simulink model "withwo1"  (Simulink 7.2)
settings: Solver=ode45  StartTime=0.0  StopTime=15  MaxStep=0.05  RelTol=1e-3
InitFcn:
  | init_withworth;
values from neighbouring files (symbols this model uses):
  L1 = 2    [init_withworth.m]    (also in init_ctyrkloub.m = 3; init_klik.m = 1.5)
  L2 = 5    [init_withworth.m]    (also in init_ctyrkloub.m; init_klik.m = v/sin(uhel3))
  omega = 0.5    [init_withworth.m]    (also in init_ctyrkloub.m = 1; init_klik.m = 5)
undefined symbols (not defined in the file or in its folder): deg, kg, m, N, rad, s
libraries: mblibv1 x14, simulink x1

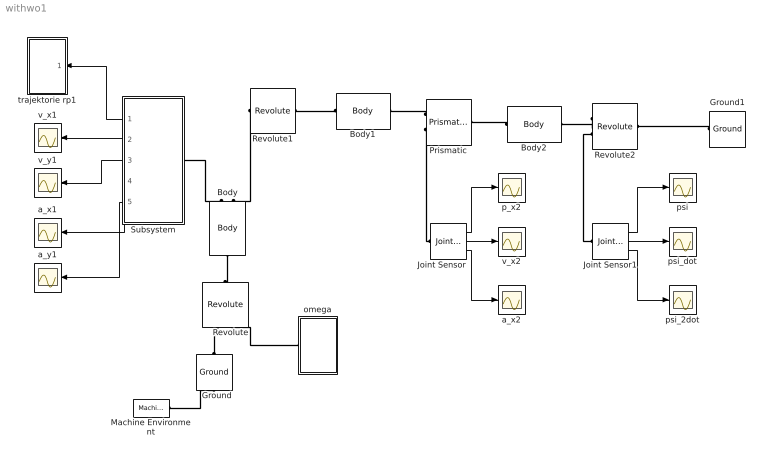
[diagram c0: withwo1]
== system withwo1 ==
  Body : mblibv1/Bodies/Body  Orientation=up  DialogController=MECH.DynMechDlgSource  PhysicalDomain=mechanical  SubClassName=Unknown  LeftPortType=workingframe  RightPortType=workingframe  LConnTagsString=CS1  RConnTagsString=CS3|CS2  UpdateFromCAD=off  DialogClass=MechanicalBodyBlock  Mass=1  MassUnits=kg  InertiaUnits=kg*m^2  Inertia=eye(3)  Shape=Cylinder  ShapeDims=[1 1]  ShapeUnits=m  ShapeUse=false  Density=1  DensityUnits=kg/m^3  DensityUse=false  GraphicsMode=MACHINE_DEFAULT  BodyColorSelMode=MACHINE_DEFAULT  BodyColor=[1 0 0]  AttachedToCS=CG  CG=Left$CG$[L1/2 0 0]$CS1$CS1$m$[0 0 pi/3]$Euler X-Y-Z$rad$WORLD$false$none  WorkingFrames=Right$CS3$[0 0 0]$CS2$CS2$m$[0 0 pi/3]$Euler X-Y-Z$rad$WORLD$true$none#Left$CS1$[0 0 0]$Adjoining$Adjoining$m$[0 0 pi/3]$Euler X-Y-Z$rad$WORLD$true$none#Right$CS2$[L1 0 0]$CS1$CS1$m$[0 0 pi/3]$Euler X-Y-Z$rad$WORLD$true$none  CGPos=[L1/2 0 0]  CGRot=[0 0 pi/3]  CS0Pos=[]  CS0Rot=[]  CS1Pos=[0 0 0]  CS1Rot=[0 0 pi/3]  CS2Pos=[L1 0 0]  CS2Rot=[0 0 pi/3]  CS3Pos=[0 0 0]  CS3Rot=[0 0 pi/3]  CS4Pos=[]  CS4Rot=[]  CS5Pos=[]  CS5Rot=[]  CS6Pos=[]  CS6Rot=[]  CS7Pos=[]  CS7Rot=[]  CS8Pos=[]  CS8Rot=[]  CS9Pos=[]  CS9Rot=[]  CS10Pos=[]  CS10Rot=[]  CS11Pos=[]  CS11Rot=[]  CS12Pos=[]  CS12Rot=[]  CS13Pos=[]  CS13Rot=[]  CS14Pos=[]  CS14Rot=[]  CS15Pos=[]  CS15Rot=[]  CS16Pos=[]  CS16Rot=[]  CS17Pos=[]  CS17Rot=[]  CS18Pos=[]  CS18Rot=[]  CS19Pos=[]  CS19Rot=[]  CS20Pos=[]  CS20Rot=[]
  Body1 : mblibv1/Bodies/Body  DialogController=MECH.DynMechDlgSource  PhysicalDomain=mechanical  SubClassName=Unknown  LeftPortType=workingframe  RightPortType=workingframe  LConnTagsString=CS1  RConnTagsString=CS2  UpdateFromCAD=off  DialogClass=MechanicalBodyBlock  Mass=1  MassUnits=kg  InertiaUnits=kg*m^2  Inertia=eye(3)  Shape=Cylinder  ShapeDims=[1 1]  ShapeUnits=m  ShapeUse=false  Density=1  DensityUnits=kg/m^3  DensityUse=false  GraphicsMode=MACHINE_DEFAULT  BodyColorSelMode=MACHINE_DEFAULT  BodyColor=[1 0 0]  AttachedToCS=CG  CG=Left$CG$[0 0 0]$CS1$CS1$m$[0 0 0]$Euler X-Y-Z$rad$CS1$false$none  WorkingFrames=Left$CS1$[0 0 0]$Adjoining$Adjoining$m$[0 0 3*pi/2]$Euler X-Y-Z$rad$Adjoining$true$none#Right$CS2$[0 0 0]$CS1$CS1$m$[0 0 0]$Euler X-Y-Z$rad$CS1$true$none  CGPos=[0 0 0]  CGRot=[0 0 0]  CS0Pos=[]  CS0Rot=[]  CS1Pos=[0 0 0]  CS1Rot=[0 0 3*pi/2]  CS2Pos=[0 0 0]  CS2Rot=[0 0 0]  CS3Pos=[]  CS3Rot=[]  CS4Pos=[]  CS4Rot=[]  CS5Pos=[]  CS5Rot=[]  CS6Pos=[]  CS6Rot=[]  CS7Pos=[]  CS7Rot=[]  CS8Pos=[]  CS8Rot=[]  CS9Pos=[]  CS9Rot=[]  CS10Pos=[]  CS10Rot=[]  CS11Pos=[]  CS11Rot=[]  CS12Pos=[]  CS12Rot=[]  CS13Pos=[]  CS13Rot=[]  CS14Pos=[]  CS14Rot=[]  CS15Pos=[]  CS15Rot=[]  CS16Pos=[]  CS16Rot=[]  CS17Pos=[]  CS17Rot=[]  CS18Pos=[]  CS18Rot=[]  CS19Pos=[]  CS19Rot=[]  CS20Pos=[]  CS20Rot=[]
  Body2 : mblibv1/Bodies/Body  DialogController=MECH.DynMechDlgSource  PhysicalDomain=mechanical  SubClassName=Unknown  LeftPortType=workingframe  RightPortType=workingframe  LConnTagsString=CS1  RConnTagsString=CS2  UpdateFromCAD=off  DialogClass=MechanicalBodyBlock  Mass=1  MassUnits=kg  InertiaUnits=kg*m^2  Inertia=eye(3)  Shape=Cylinder  ShapeDims=[1 1]  ShapeUnits=m  ShapeUse=false  Density=1  DensityUnits=kg/m^3  DensityUse=false  GraphicsMode=MACHINE_DEFAULT  BodyColorSelMode=MACHINE_DEFAULT  BodyColor=[1 0 0]  AttachedToCS=CG  CG=Left$CG$[L2/2 0 0]$CS1$CS1$m$[0 0 0]$Euler X-Y-Z$deg$CS1$false$none  WorkingFrames=Left$CS3$[-L2/2 0 0]$CS1$CS1$m$[0 0 0]$Euler X-Y-Z$deg$CS1$false$none#Left$CS1$[0 0 0]$Adjoining$Adjoining$m$[0 0 0]$Euler X-Y-Z$deg$Adjoining$true$none#Right$CS2$[L2 0 0]$CS1$CS1$m$[0 0 0]$Euler X-Y-Z$deg$CS1$true$none  CGPos=[L2/2 0 0]  CGRot=[0 0 0]  CS0Pos=[]  CS0Rot=[]  CS1Pos=[0 0 0]  CS1Rot=[0 0 0]  CS2Pos=[L2 0 0]  CS2Rot=[0 0 0]  CS3Pos=[-L2/2 0 0]  CS3Rot=[0 0 0]  CS4Pos=[]  CS4Rot=[]  CS5Pos=[]  CS5Rot=[]  CS6Pos=[]  CS6Rot=[]  CS7Pos=[]  CS7Rot=[]  CS8Pos=[]  CS8Rot=[]  CS9Pos=[]  CS9Rot=[]  CS10Pos=[]  CS10Rot=[]  CS11Pos=[]  CS11Rot=[]  CS12Pos=[]  CS12Rot=[]  CS13Pos=[]  CS13Rot=[]  CS14Pos=[]  CS14Rot=[]  CS15Pos=[]  CS15Rot=[]  CS16Pos=[]  CS16Rot=[]  CS17Pos=[]  CS17Rot=[]  CS18Pos=[]  CS18Rot=[]  CS19Pos=[]  CS19Rot=[]  CS20Pos=[]  CS20Rot=[]
  Ground : mblibv1/Bodies/Ground  Orientation=up  DialogController=MECH.DynMechDlgSource  SystemSampleTime=-1  UpdateFromCAD=off  LeftPortType=env  RightPortType=workingframe  PhysicalDomain=Mechanical  DialogClass=GroundBlock  CoordPosition=[0 0 0]  CoordPositionUnits=m  StateVectorMgrId=2  MachineId=[3 0]  ShowEnvPort=on
  Ground1 : mblibv1/Bodies/Ground  Orientation=left  DialogController=MECH.DynMechDlgSource  SystemSampleTime=-1  UpdateFromCAD=off  LeftPortType=env  RightPortType=workingframe  PhysicalDomain=Mechanical  DialogClass=GroundBlock  CoordPosition=[L1*cos(pi/3)+L2*cos(pi/6) L1*sin(pi/3)-L2*sin(pi/6) 0]  CoordPositionUnits=m  StateVectorMgrId=-1  MachineId=[0 0]  ShowEnvPort=off
  Joint Sensor : mblibv1/Sensors &  Actuators/Joint Sensor  DialogController=MECH.DynMechDlgSource  SystemSampleTime=-1  UpdateFromCAD=off  PhysicalDomain=Mechanical  PortType=blob  Muxed=off  Pose=off  Angle=on  AngleUnits=deg  ArcVelocity=off  ArcVelocityUnits=deg/s  ArcAcceleration=off  ArcAccelerationUnits=deg/s^2  CoordPosition=on  CoordPositionUnits=m  Velocity=on  VelocityUnits=m/s  Acceleration=on  AccelerationUnits=m/s^2  Quaternion=on  QuaternionDT=off  QuaternionDDT=off  QuaternionUnits=off  OutputVector=[1]  ActiveIO=on  Width=3  DialogClass=MechanicalSensorBlock  Primitive=P1  Force=off  ForceUnits=N  Torque=off  TorqueUnits=N*m  ReferenceFrame=Absolute (World)  ReactionSensedSide=Base  ReactionReferenceFrame=Absolute (World)  ReactionForce=off  ReactionForceUnits=N  ReactionMoment=off  ReactionMomentUnits=N*m
  Joint Sensor1 : mblibv1/Sensors &  Actuators/Joint Sensor  DialogController=MECH.DynMechDlgSource  SystemSampleTime=-1  UpdateFromCAD=off  PhysicalDomain=Mechanical  PortType=blob  Muxed=off  Pose=off  Angle=on  AngleUnits=rad  ArcVelocity=on  ArcVelocityUnits=rad/s  ArcAcceleration=on  ArcAccelerationUnits=rad/s^2  CoordPosition=on  CoordPositionUnits=m  Velocity=on  VelocityUnits=m/s  Acceleration=on  AccelerationUnits=m/s^2  Quaternion=on  QuaternionDT=off  QuaternionDDT=off  QuaternionUnits=off  OutputVector=[1]  ActiveIO=on  Width=3  DialogClass=MechanicalSensorBlock  Primitive=R1  Force=off  ForceUnits=N  Torque=off  TorqueUnits=N*m  ReferenceFrame=Absolute (World)  ReactionSensedSide=Base  ReactionReferenceFrame=Absolute (World)  ReactionForce=off  ReactionForceUnits=N  ReactionMoment=off  ReactionMomentUnits=N*m
  Machine Environment : mblibv1/Bodies/Machine Environment  DialogController=MECH.DialogSource  SystemSampleTime=-1  PortType=env  PhysicalDomain=Mechanical  DialogTemplateClass=MECH.MachineEnvironment  SyncWhenCopied=off  Gravity=[0 -9.81 0]  GravityUnits=m/s^2  GravityAsSignal=off  Dimensionality=Auto-detect  AnalysisType=Kinematics  LinearAssemblyTolerance=1e-3  LinearAssemblyToleranceUnits=m  AngularAssemblyTolerance=1e-3  AngularAssemblyToleranceUnits=rad  ConstraintSolverType=Stabilizing  ConstraintRelTolerance=1e-4  ConstraintAbsTolerance=1e-4  UseRobustSingularityHandling=off  RedundancyAnalysisToleranceType=Automatically select tolerance  RedundancyAnalysisTolerance=1e-14  StatePerturbationType=Fixed  PerturbationSize=1e-5  VisualizeMachine=on  BodyVisualizationType=Use model default body geometries  BodyColorSelMode=Use model default  DefaultBodyColor=[1 0 0]
  Prismatic : mblibv1/Joints/Prismatic  DialogController=MECH.DynMechDlgSource  PhysicalDomain=mechanical  SubClassName=Unknown  LeftPortType=blob  RightPortType=blob  LConnTagsString=__newl0|SA1  RConnTagsString=__newr0  UpdateFromCAD=off  NumSAPorts=1  CutJoint=off  MarkAsCut=off  Primitives=prismatic  PrimitiveProps=P1$Base$[-1 0 0]$prismatic  DialogClass=JointBlock  P1Axis=[-1 0 0]
  Revolute : mblibv1/Joints/Revolute  Orientation=up  DialogController=MECH.DynMechDlgSource  PhysicalDomain=mechanical  SubClassName=Unknown  LeftPortType=blob  RightPortType=blob  LConnTagsString=__newl0|SA1  RConnTagsString=__newr0  UpdateFromCAD=off  NumSAPorts=1  CutJoint=off  MarkAsCut=off  Primitives=prismatic  PrimitiveProps=R1$World$[0 0 1]$revolute  DialogClass=JointBlock  R1Axis=[0 0 1]
  Revolute1 : mblibv1/Joints/Revolute  DialogController=MECH.DynMechDlgSource  PhysicalDomain=mechanical  SubClassName=Unknown  LeftPortType=blob  RightPortType=blob  LConnTagsString=__newl0  RConnTagsString=__newr0  UpdateFromCAD=off  NumSAPorts=0  CutJoint=off  MarkAsCut=off  Primitives=prismatic  PrimitiveProps=R1$WORLD$[0 0 1]$revolute  DialogClass=JointBlock  R1Axis=[0 0 1]
  Revolute2 : mblibv1/Joints/Revolute  DialogController=MECH.DynMechDlgSource  PhysicalDomain=mechanical  SubClassName=Unknown  LeftPortType=blob  RightPortType=blob  LConnTagsString=__newl0|SA1  RConnTagsString=__newr0  UpdateFromCAD=off  NumSAPorts=1  CutJoint=off  MarkAsCut=off  Primitives=prismatic  PrimitiveProps=R1$World$[0 0 1]$revolute  DialogClass=JointBlock  R1Axis=[0 0 1]
  Subsystem : Subsystem  Orientation=left
  a_x1 : Scope
  a_x2 : Scope
  a_y1 : Scope
  omega : Subsystem  Orientation=left
  p_x2 : Scope
  psi : Scope
  psi_2dot : Scope
  psi_dot : Scope
  trajektorie rp1 : Subsystem  Orientation=left
  v_x1 : Scope
  v_x2 : Scope
  v_y1 : Scope
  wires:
  Joint Sensor/1 -> p_x2/1
  Joint Sensor/2 -> v_x2/1
  Joint Sensor/3 -> a_x2/1
  Subsystem/1(Out1) -> trajektorie rp1/1(In1)
  Subsystem/2(Out2) -> v_x1/1
  Subsystem/3(Out3) -> v_y1/1
  Subsystem/4(Out4) -> a_x1/1
  Subsystem/5(Out5) -> a_y1/1
  Joint Sensor1/1 -> psi/1
  Joint Sensor1/2 -> psi_dot/1
  Joint Sensor1/3 -> psi_2dot/1
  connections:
  Ground/RConn1 -- Revolute/LConn1
  Body/LConn1 -- Revolute/RConn1
  Revolute1/LConn1 -- Body/RConn2
  Body1/LConn1 -- Revolute1/RConn1
  Prismatic/LConn1 -- Body1/RConn1
  Body2/LConn1 -- Prismatic/RConn1
  Ground1/RConn1 -- Revolute2/RConn1
  Revolute2/LConn1 -- Body2/RConn1
  Subsystem/LConn1 -- Body/RConn1
  omega/RConn1 -- Revolute/LConn2
  Joint Sensor/LConn1 -- Prismatic/LConn2
  Machine Environment/RConn1 -- Ground/LConn1
  Joint Sensor1/LConn1 -- Revolute2/LConn2

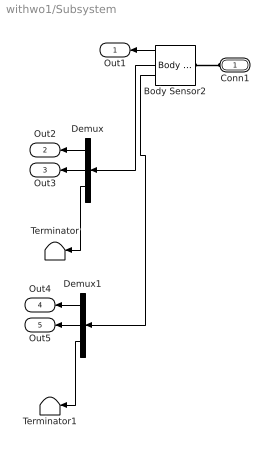
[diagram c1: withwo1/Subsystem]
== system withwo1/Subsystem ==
  Body Sensor2 : mblibv1/Sensors &  Actuators/Body Sensor  Orientation=left  DialogController=MECH.DynMechDlgSource  SystemSampleTime=-1  UpdateFromCAD=off  PhysicalDomain=Mechanical  PortType=blob  Muxed=off  Pose=off  Angle=on  AngleUnits=deg  ArcVelocity=off  ArcVelocityUnits=deg/s  ArcAcceleration=off  ArcAccelerationUnits=deg/s^2  CoordPosition=on  CoordPositionUnits=m  Velocity=on  VelocityUnits=m/s  Acceleration=on  AccelerationUnits=m/s^2  Quaternion=on  QuaternionDT=off  QuaternionDDT=off  QuaternionUnits=off  OutputVector=[1]  ActiveIO=on  Width=9  DialogClass=MechanicalSensorBlock  ReferenceFrame=Absolute (World)
  Demux : Demux  Orientation=left  Outputs=3
  Demux1 : Demux  Orientation=left  Outputs=3
  Terminator : Terminator
  Terminator1 : Terminator
  Conn1 : PMIOPort  Orientation=left  Port=1  Side=Left
  Out1 : Outport  Orientation=left
  Out2 : Outport  Orientation=left  Port=2
  Out3 : Outport  Orientation=left  Port=3
  Out4 : Outport  Orientation=left  Port=4
  Out5 : Outport  Orientation=left  Port=5
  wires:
  Demux/3 -> Terminator/1
  Body Sensor2/2 -> Demux/1
  Demux1/3 -> Terminator1/1
  Body Sensor2/3 -> Demux1/1
  Body Sensor2/1 -> Out1/1
  Demux/1 -> Out2/1
  Demux/2 -> Out3/1
  Demux1/1 -> Out4/1
  Demux1/2 -> Out5/1
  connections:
  Conn1/RConn1 -- Body Sensor2/LConn1

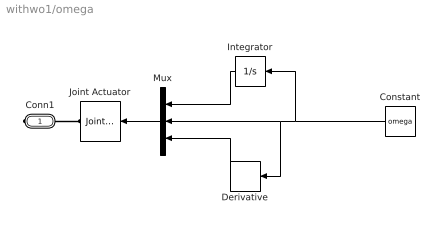
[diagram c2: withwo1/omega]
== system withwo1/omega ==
  Constant : Constant  Orientation=left  Value=omega  OutDataType=sfix(16)  OutScaling=2^0
  Derivative : Derivative  Orientation=left
  Integrator : Integrator  Orientation=left
  Joint Actuator : mblibv1/Sensors &  Actuators/Joint Actuator  Orientation=left  DialogController=MECH.DynMechDlgSource  SystemSampleTime=-1  UpdateFromCAD=off  PhysicalDomain=Mechanical  PortType=blob  ActuationStyle=Motion  AngleUnits=rad  ArcVelocityUnits=rad/s  ArcAccelerationUnits=rad/s^2  CoordPositionUnits=m  VelocityUnits=m/s  AccelerationUnits=m/s^2  ForceUnits=N  TorqueUnits=N*m  ActiveIO=on  Width=3  DialogClass=MechanicalActuatorBlock  Primitive=R1  ReferenceFrame=Absolute (World)
  Mux : Mux  Orientation=left  Inputs=3
  Conn1 : PMIOPort  Port=1  Side=Right
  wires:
  Constant/1 -> Derivative/1, Mux/2, Integrator/1
  Mux/1 -> Joint Actuator/1
  Integrator/1 -> Mux/1
  Derivative/1 -> Mux/3
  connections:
  Conn1/RConn1 -- Joint Actuator/RConn1

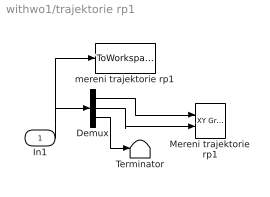
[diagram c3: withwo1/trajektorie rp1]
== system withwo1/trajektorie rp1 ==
  In1 : Inport
  Demux : Demux  Outputs=3
  Mereni trajektorie rp1 : simulink/Sinks/XY Graph  SystemSampleTime=-1  xmin=-3.3  xmax=3.3  ymin=-2.5  ymax=2.5  st=-1
  Terminator : Terminator
  mereni trajektorie rp1 : ToWorkspace  VariableName=rot  SampleTime=-1  SaveFormat=Array
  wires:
  Demux/1 -> Mereni trajektorie rp1/1
  Demux/2 -> Mereni trajektorie rp1/2
  Demux/3 -> Terminator/1
  In1/1 -> mereni trajektorie rp1/1, Demux/1
